// TwinCAT 3 PLC project Untitled1
// ProgramVersion: 3.1.4022.2
// libraries:
//   Tc2_Standard, * (Beckhoff Automation GmbH)
//   Tc2_System, * (Beckhoff Automation GmbH)
//   Tc2_Utilities, * (Beckhoff Automation GmbH)
//   Tc3_Module, * (Beckhoff Automation GmbH)
// project tree:
//   / CsvTask.TcTTO, PlcTask.TcTTO
//   DUTs/ ST_Buffer.TcDUT, T_Buffer.TcDUT
//   FBs/ FB_CSV.TcPOU, FB_Writer.TcPOU
//   GVLs/ GVL.TcGVL
//   POUs/ FastTask.TcPOU, MAIN.TcPOU
// real-time tasks:
//   TASK PlcTask: cycle T#10ms, priority 20, ADS port 350
//   TASK CsvTask: cycle T#1ms, priority 1, ADS port 351

CONFIGURATION Untitled1
    RESOURCE PLC ON TwinCAT3
        TASK CsvTask(INTERVAL := T#1ms, PRIORITY := 1);
        TASK PlcTask(INTERVAL := T#10ms, PRIORITY := 20);
        PROGRAM FastTask WITH CsvTask : FastTask;
        PROGRAM MAIN WITH PlcTask : MAIN;
    END_RESOURCE
END_CONFIGURATION

// ---- DUTs/ST_Buffer.TcDUT
TYPE ST_Buffer :
STRUCT
	bFull 		: BOOL;
	sPath		: STRING;
	aBuffer 	: ARRAY[0..MAX_CSV_ROWS, 0..MAX_CSV_COLUMNS ] OF STRING(MAX_CSV_FIELD_LENGTH) ;
	fbWriter 	: FB_Writer;
END_STRUCT
END_TYPE

// ---- DUTs/T_Buffer.TcDUT
TYPE T_Buffer: ARRAY[0..MAX_CSV_ROWS, 0..MAX_CSV_COLUMNS ] OF STRING(MAX_CSV_FIELD_LENGTH); (* [] (* TODESC *) *)
END_TYPE

// ---- GVLs/GVL.TcGVL
VAR_GLOBAL
	iData1:REAL;
	iData2:INT;
	iData3:STRING;
	
	iData4: WSTRING;
END_VAR
 

VAR_GLOBAL
	gCSV_Buffer: ARRAY[0..MAX_CSV_RING_BUFFER] OF ST_Buffer;
END_VAR

VAR_GLOBAL CONSTANT
	MAX_CSV_ROWS 			: UDINT := 3000;(*最大行数(任务周期为20ms)即10分钟的buffer*)
	MAX_CSV_COLUMNS 		: UDINT := 100;(*最大列数*)
	MAX_CSV_FIELD_LENGTH	: UDINT := 35;(*每个字段的字符长度*)
	MAX_CSV_RING_BUFFER		: UDINT := 4;
END_VAR

// ---- POUs/FastTask.TcPOU
PROGRAM FastTask
VAR
	_iBuffer: UDINT := 0;
END_VAR

FOR _iBuffer := 0 TO MAX_CSV_RING_BUFFER BY 1 DO
	IF gCSV_Buffer[_iBuffer].bFull THEN
		gCSV_Buffer[_iBuffer].fbWriter(bWrite:= gCSV_Buffer[_iBuffer].bFull,sFileName:=gCSV_Buffer[_iBuffer].sPath, pBuffer :=ADR(gCSV_Buffer[_iBuffer].aBuffer));
		gCSV_Buffer[_iBuffer].bFull := gCSV_Buffer[_iBuffer].fbWriter.bBusy;
	END_IF
END_FOR

END_PROGRAM

// ---- POUs/MAIN.TcPOU
PROGRAM MAIN
VAR 
	fbCSV: FB_CSV;
	
	{ attribute 'TcEncoding' := 'UTF-8'}
	sTemp: STRING; 
END_VAR

VAR CONSTANT
	ci_DecimalPlaces: USINT:= 3; (*保留有效数字 *)
END_VAR

IF fbCSV.bRingBufferFull THEN
	RETURN;
END_IF


iData1 := iData1 + 0.001;
iData2 := iData2 + 1;
iData3 := 'Test';
iData4 := "倍福中国";
 
Wstring_to_UTF8(ADR(sTemp), ADR(iData4),SIZEOF(iData4));


fbCSV.pRowData[1] := LREAL_TO_FMTSTR(iData1, ci_DecimalPlaces, TRUE); 
fbCSV.pRowData[2] :=INT_TO_STRING(iData2); 
fbCSV.pRowData[3] := iData3;
fbCSV.pRowData[4] := sTemp;


fbCSV(sPath:= 'D:');

END_PROGRAM

// ---- FBs/FB_CSV.TcPOU
FUNCTION_BLOCK FB_CSV
VAR_INPUT
	sPath: STRING(255);
	pRowData: ARRAY[1..MAX_CSV_COLUMNS] OF STRING(MAX_CSV_FIELD_LENGTH);
END_VAR
VAR_OUTPUT
	bRingBufferFull: BOOL;
END_VAR
VAR
	fbSysTime	: 	GETSYSTEMTIME;
	tFileTime	:	T_FILETIME;  
	
	_tNow		:	TIMESTRUCT; 
	   
	_iRowIndex: UDINT := 2; (*第1行存储字段名，2行存储PLC变量名*) 
	
	_iRingBuffer	: DWORD 	:= 0;
	
	fbFormat 	: 	FB_FormatString;
	_sPathFormat	: T_MaxString := '%s\%d__%d_%d_%d_%d_%d.csv';   
	_index: UDINT;
END_VAR
 
VAR CONSTANT
	cs_Seperator: STRING[1]:= ';'; (*CSV字段分隔符*)
	cs_CarriageReturn: STRING[2]:= '$R$N'; (*回车换行符*)
	
	MAX_BEFFER_SIZE:UINT := 8192;(*每条ADS写命令写下去的内存大小*)
END_VAR

fbSysTime(timeLoDW=>tFileTime.dwLowDateTime , timeHiDW=> tFileTime.dwHighDateTime);

_tNow := FILETIME_TO_SYSTEMTIME(tFileTime);
IF _tNow.wYear = 0 THEN
	RETURN;
END_IF
  
A_RowData();

_iRowIndex := _iRowIndex + 1;
IF _iRowIndex >= MAX_CSV_ROWS THEN 
	A_Header();	 	 
	gCSV_Buffer[_iRingBuffer].bFull := TRUE;
	
	fbFormat( 	sFormat := _sPathFormat ,
			 	arg1 := F_STRING(sPath),   arg2 := F_WORD(_tNow.wYear), arg3 := F_WORD(_tNow.wMonth), 
				arg4 := F_WORD(_tNow.wDay), arg5 := F_WORD(_tNow.wHour),arg6 := F_WORD(_tNow.wMinute),
			    arg7 := F_WORD(_tNow.wSecond),  sOut => gCSV_Buffer[_iRingBuffer].sPath);
				
	_iRingBuffer := _iRingBuffer + 1;
	IF _iRingBuffer > MAX_CSV_RING_BUFFER THEN
		IF gCSV_Buffer[_iRingBuffer].bFull THEN
			bRingBufferFull := TRUE;
		END_IF
		_iRingBuffer := 0; 
	END_IF
	_iRowIndex := 2;
END_IF

ACTION A_Header:
(*第一行 字段名称*) 
gCSV_Buffer[_iRingBuffer].aBuffer[ 0, 0] := 'WindSpeed';
gCSV_Buffer[_iRingBuffer].aBuffer[ 0, 1] := 'WindVane';
gCSV_Buffer[_iRingBuffer].aBuffer[ 0, 2] := 'TimeStampPLC3'; 
gCSV_Buffer[_iRingBuffer].aBuffer[ 0, 3] := 'TimeStampPLC4'; 
gCSV_Buffer[_iRingBuffer].aBuffer[ 0, 4] := 'TimeStampPLC5'; 

(*第二行 PLC变量名*)
gCSV_Buffer[_iRingBuffer].aBuffer[ 1, 0] := 'MAIN.var1';
gCSV_Buffer[_iRingBuffer].aBuffer[ 1, 1] := 'MAIN.var2'; 
gCSV_Buffer[_iRingBuffer].aBuffer[ 1, 2] := 'MAIN.var3'; 
gCSV_Buffer[_iRingBuffer].aBuffer[ 1, 3] := 'MAIN.var4'; 
gCSV_Buffer[_iRingBuffer].aBuffer[ 1, 4] := 'MAIN.var5';
END_ACTION

ACTION A_RowData:

(*数据行 从第三行开始*)


gCSV_Buffer[_iRingBuffer].aBuffer[_iRowIndex,0] := SYSTEMTIME_TO_STRING(_tNow);(*第二行第一列*)

FOR _index :=1 TO MAX_CSV_COLUMNS DO 
	gCSV_Buffer[_iRingBuffer].aBuffer[_iRowIndex,_index] := pRowData[_index];
END_FOR
END_ACTION

END_FUNCTION_BLOCK

// ---- FBs/FB_Writer.TcPOU
FUNCTION_BLOCK FB_Writer
VAR_INPUT
	bWrite		: BOOL;		(* Rising edge starts program execution*)
	sNetId		: T_AmsNetId := '';	(* TwinCAT system network address *)
	sFileName	: T_MaxString;		(*  := 'HardDisk\TextModeGen.csv' CSV destination file path and name*) 
	pBuffer		: POINTER TO T_Buffer;
END_VAR
VAR_OUTPUT
	bBusy: BOOL; 
	bError			: BOOL;
	nErrId			: UDINT;
END_VAR
VAR  
	fbFileOpen	: FB_FileOpen;(* Opens file *)
	fbFileClose	: FB_FileClose;(* Closes file *)
	fbAdsRdWrt	: FW_AdsRdWrt := ( nPort := AMSPORT_R3_SYSSERV, nIdxGrp := SYSTEMSERVICE_FPUTS, cbReadLen := 0, pReadBuff := 0 );	(* Writes one record (line) *)

 	_hFile			: UINT		:= 0;(* File handle of the source file *)
	_iStep			: DWORD 	:= 0;

	_iLen1: UDINT;
	_iLen2: UDINT;
	
	_iRow: UDINT;
	_iLastRow: UDINT;
	
	_iCol: UDINT;
	_iLastCol: UDINT;
	
	_iOffset: UDINT;
	
	_iCpy: UDINT;
	_pBuffer: PVOID;
	_sBuffer: STRING(MAX_BEFFER_SIZE);
END_VAR
 
VAR CONSTANT
	cs_Seperator: STRING[1]:= ';'; (*CSV字段分隔符*)
	cs_CarriageReturn: STRING[2]:= '$R$N'; (*回车换行符*)
	
	MAX_BEFFER_SIZE:UINT := 8192;(*每条ADS写命令写下去的内存大小*)
END_VAR

CASE _iStep OF
	0:	(* Wait for rising edge at bWrite variable *)
		IF bWrite THEN
			bWrite 		:= FALSE;
			bBusy 		:= TRUE;
			bError		:= FALSE;
			nErrId		:= 0;
			_hFile		:= 0; 
			_iStep 		:= 1;
			_iLastRow 	:= 0;
			_iLastCol   := 0;
		END_IF

	1:	(* Open source file *)
		fbFileOpen(  bExecute := FALSE  );
		fbFileOpen( 	sNetId := sNetId, sPathName := sFileName, nMode := FOPEN_MODEWRITE OR FOPEN_MODETEXT,(* Open file in TEXT mode! *)
						ePath := PATH_GENERIC, bExecute := TRUE );
		_iStep := 2;

	2:(* Wait until open not busy *)
		fbFileOpen( bExecute := FALSE, bError => bError, nErrID => nErrID, hFile => _hFile );
		IF NOT fbFileOpen.bBusy THEN
			IF NOT fbFileOpen.bError THEN
				_iStep := 3;
			ELSE(* Error: file not found? *)
				_iStep := 100;
			END_IF
		END_IF

	3:(* Convert one PLC record to CSV format *) 
		MEMSET(ADR(_sBuffer),0,MAX_BEFFER_SIZE);
		_iOffset := 0;
		_iCpy := 0;
		_pBuffer := ADR(_sBuffer);
		FOR _iRow := _iLastRow TO MAX_CSV_ROWS BY 1 DO
			FOR _iCol := _iLastCol TO MAX_CSV_COLUMNS BY 1 DO 
				_iLen1 := LEN(pBuffer^[ _iRow, _iCol]);
				_iLen2 := LEN(cs_Seperator); 
				IF (_iOffset + _iLen1 + _iLen2 + 1) < MAX_BEFFER_SIZE THEN 
					_iCpy := FW_MemCpy(_pBuffer + _iOffset, ADR(pBuffer^[ _iRow, _iCol]), _iLen1);
					_iOffset := _iOffset + _iCpy;
					IF  _iCol < MAX_CSV_COLUMNS THEN
						_iCpy := FW_MemCpy(_pBuffer + _iOffset, ADR(cs_Seperator), _iLen2);
						_iOffset := _iOffset + _iCpy;
					END_IF
				ELSE
					_iLastRow := _iRow;
					_iLastCol := _iCol;
					_iStep := 4;(* Write record to the file *)
					RETURN;	
				END_IF
			END_FOR 
			_iLen2 := LEN(cs_CarriageReturn); 
			_iCpy:= FW_MemCpy(_pBuffer + _iOffset, ADR(cs_CarriageReturn), _iLen2);
			_iOffset := _iOffset + _iCpy;
			_iLastCol := 0;
		END_FOR 
		_iStep := 4;(* Write record to the file *) 
	4:	(* Write single text line *) 
		fbAdsRdWrt( bExecute := FALSE ); 
		fbAdsRdWrt( sNetId := sNetId, nIdxOffs := _hFile, cbWriteLen := _iOffset + 1(*inclusive terminating NULL*), pWriteBuff := ADR(_sBuffer),
			bExecute := TRUE, tTimeout := DEFAULT_ADS_TIMEOUT, bBusy=>bBusy, bError=>bError, nErrID=>nErrID );
		_iStep := 5;

	5:(* Wait until write not busy *)
		fbAdsRdWrt( bExecute := FALSE, bError => bError, nErrID => nErrID );
		IF NOT fbAdsRdWrt.bBusy THEN
			IF NOT fbAdsRdWrt.bError THEN 
				_iStep := 3;(* Write next record *)
				IF _iRow >= MAX_CSV_ROWS THEN
					_iStep := 10;
				END_IF
			ELSE(* Error *)
				_iStep := 100;
			END_IF
		END_IF

	10:	(* Close source file *)
		fbFileClose( bExecute := FALSE );
		fbFileClose( sNetId := sNetId, hFile := _hFile, bExecute := TRUE );
		_iStep := 11;

	11:(* Wait until close not busy *)
		fbFileClose( bExecute := FALSE, bError => bError, nErrID => nErrID );
		IF ( NOT fbFileClose.bBusy ) THEN
			_hFile := 0;
			_iStep := 100;
		END_IF

	100: (* Error or ready step => cleanup *)
		IF ( _hFile <> 0 ) THEN
			_iStep := 10; (* Close the source file *)
		ELSE
			bBusy := FALSE;
			_iStep := 0;	(* Ready *) 
		END_IF

END_CASE

END_FUNCTION_BLOCK
